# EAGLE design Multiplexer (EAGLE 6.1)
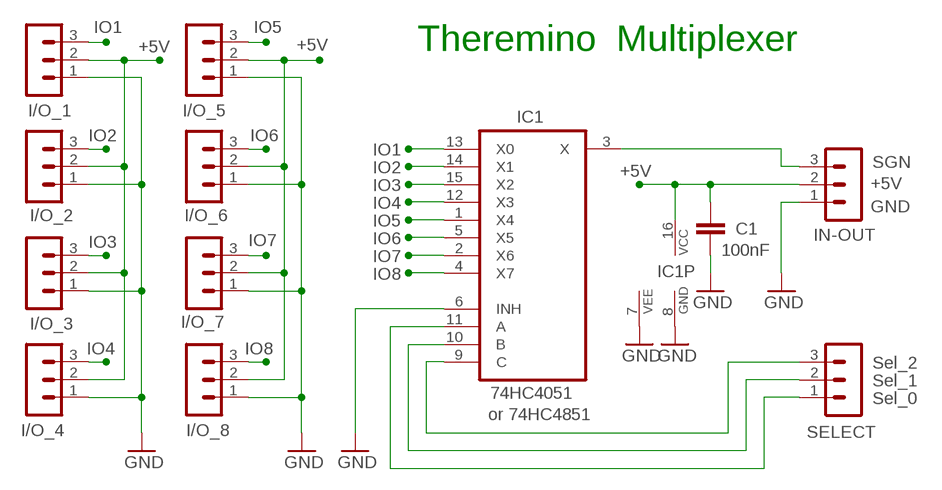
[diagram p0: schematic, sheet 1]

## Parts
C1  100nF  C-EU025-025X050  [C025-025X050]
I/O_1  MA03-1L3  [MA03-1_L3]
I/O_2  MA03-1L3  [MA03-1_L3]
I/O_3  MA03-1L3  [MA03-1_L3]
I/O_4  MA03-1L3  [MA03-1_L3]
I/O_5  MA03-1L3  [MA03-1_L3]
I/O_6  MA03-1L3  [MA03-1_L3]
I/O_7  MA03-1L3  [MA03-1_L3]
I/O_8  MA03-1L3  [MA03-1_L3]
IC1  74HC4051  4051N  [DIL16]
IN-OUT  MA03-1L3  [MA03-1_L3]
SELECT  MA03-1L3  [MA03-1_L3]

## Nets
+5V: C1.1 I/O_1.2 I/O_2.2 I/O_3.2 I/O_4.2 I/O_5.2 I/O_6.2 I/O_7.2 I/O_8.2 IC1.16(VCC) IN-OUT.2
GND: C1.2 I/O_1.1 I/O_2.1 I/O_3.1 I/O_4.1 I/O_5.1 I/O_6.1 I/O_7.1 I/O_8.1 IC1.6(INH) IC1.7(VEE) IC1.8(GND) IN-OUT.1
IO1: I/O_1.3 IC1.13(X0)
IO2: I/O_2.3 IC1.14(X1)
IO3: I/O_3.3 IC1.15(X2)
IO4: I/O_4.3 IC1.12(X3)
IO5: I/O_5.3 IC1.1(X4)
IO6: I/O_6.3 IC1.5(X5)
IO7: I/O_7.3 IC1.2(X6)
IO8: I/O_8.3 IC1.4(X7)
N$1: IC1.3(X) IN-OUT.3
N$2: IC1.11(A) SELECT.1
N$3: IC1.10(B) SELECT.2
N$4: IC1.9(C) SELECT.3

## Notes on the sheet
- Theremino | Multiplexer
- SGN
- +5V
- GND
- Sel_2
- Sel_1
- Sel_0
- or 74HC4851

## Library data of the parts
C1 = 00-LIVIO:C-EU: CAPACITOR, European symbol
I/O_1-I/O_8 IN-OUT SELECT = 03-con-lstb-M:MA03-1: PIN HEADER
IC1 = 00-LIVIO:4051: 8-channel ANALOG MULTIPLEXER

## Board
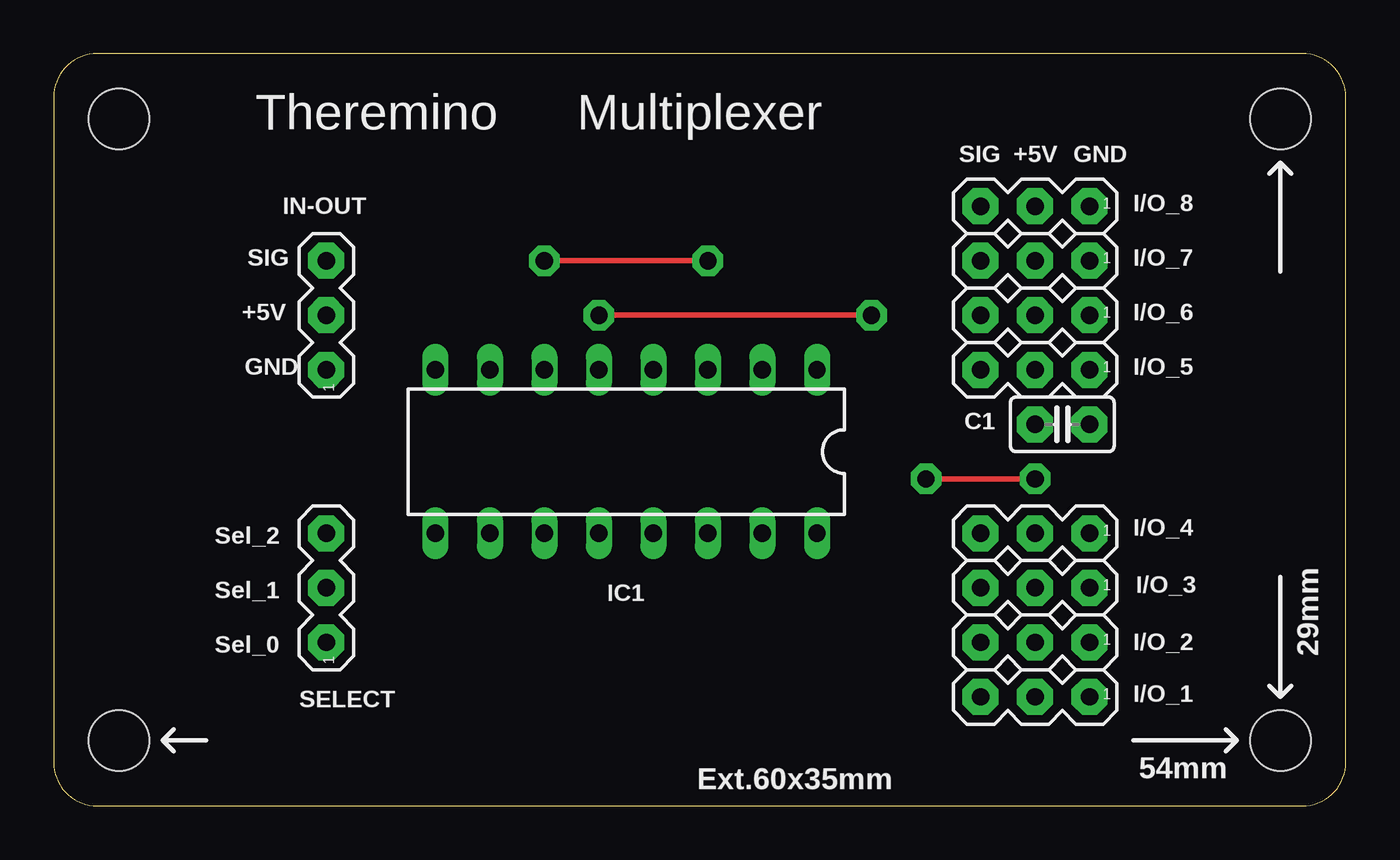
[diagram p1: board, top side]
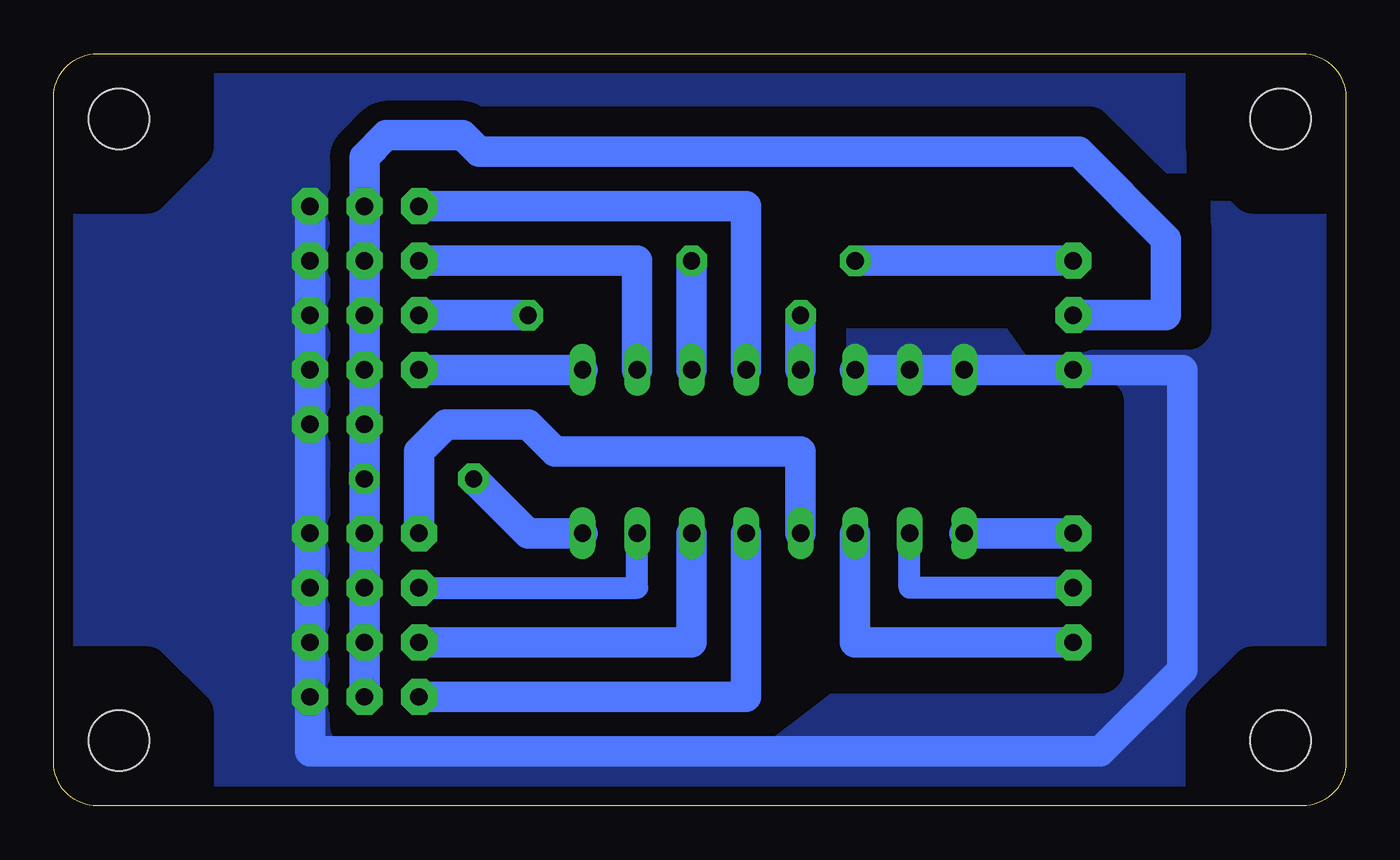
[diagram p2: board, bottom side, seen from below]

Size 60.2 x 35.05 mm. Coordinates in mm from the lower left corner, seen from the top.
Outline: 2.03,0 58.17,0 arc90 60.2,2.03 60.2,33.02 arc90 58.17,35.05 2.03,35.05 arc90 0,33.02 0,2.03 arc90 2.03,0
Copper layers (1*16): Top 0.035mm / dielectric 1.5mm / Bottom 0.035mm
Design rules: minimum track width 10mil, minimum drill 31mil, track to track 31mil, track to pad 31mil, pad to pad 31mil, via to via 31mil, smd to smd 31mil, copper to edge 31mil, drill to drill 8mil, minimum pad ring 5mil, minimum via ring 8mil, stop-mask expansion 4mil, vias tented up to drill 0mil, thermal gap 47mil
Holes 2.8 mm at 57.15,32 57.15,3.05 3.05,32 3.05,3.05
bRestrict: 23 lines

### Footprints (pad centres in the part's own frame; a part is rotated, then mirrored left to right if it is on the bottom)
C025-025X050 = drill 0.813 pad 1.676 octagon: 1 -1.27,0; 2 1.27,0
MA03-1_L3 = drill 0.813 pad 1.676 octagon: 1 -2.54,0; 2 0,0; 3 2.54,0
DIL16 = drill 0.813 long: 1 -8.89,-3.81; 2 -6.35,-3.81; 3 -3.81,-3.81; 4 -1.27,-3.81; 5 1.27,-3.81; 6 3.81,-3.81; 7 6.35,-3.81; 8 8.89,-3.81; 9 8.89,3.81; 10 6.35,3.81; 11 3.81,3.81; 12 1.27,3.81; 13 -1.27,3.81; 14 -3.81,3.81; 15 -6.35,3.81; 16 -8.89,3.81

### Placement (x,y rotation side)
C1  46.99,17.78 0 top
I/O_1  45.72,5.08 180 top
I/O_2  45.72,7.62 180 top
I/O_3  45.72,10.16 180 top
I/O_4  45.72,12.7 180 top
I/O_5  45.72,20.32 180 top
I/O_6  45.72,22.86 180 top
I/O_7  45.72,25.4 180 top
I/O_8  45.72,27.94 180 top
IC1  26.67,16.51 180 top
IN-OUT  12.7,22.86 90 top
SELECT  12.7,10.16 90 top

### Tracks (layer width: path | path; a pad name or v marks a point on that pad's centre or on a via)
+5V  (via drill 0.8 pad 1.42)
  Top 0.254: v40.64,15.24 v45.72,15.24
  Bottom 1.422: IN-OUT.2 8.38,22.86 8.38,26.42 12.45,30.48 40.39,30.48 41.15,31.24 44.7,31.24 45.72,30.23 I/O_8.2 I/O_7.2 I/O_6.2 I/O_5.2 C1.1 v45.72,15.24 I/O_4.2 I/O_3.2 I/O_2.2 I/O_1.2 | IC1.16 38.1,12.7 v40.64,15.24
GND
  Bottom 1.422: IN-OUT.1 IC1.8 IC1.7 IC1.6 IN-OUT.1 | I/O_1.1 I/O_2.1 I/O_3.1 I/O_4.1 C1.2 | I/O_8.1 I/O_7.1 I/O_6.1 I/O_5.1 C1.2 | C1.2 48.26,2.54 11.43,2.54 7.62,6.35 7.62,20.32 IN-OUT.1
  pour Bottom (isolate 0.9, no thermals): -1,-1 61.2,-1 61.2,36.05 -1,36.05
IO1
  Bottom 1.422: I/O_1.3 27.94,5.08 IC1.13
IO2
  Bottom 1.422: IC1.14 30.48,7.62 I/O_2.3
IO3
  Bottom 1.016: I/O_3.3 33.02,10.16 IC1.15
IO4
  Bottom 1.422: I/O_4.3 43.18,16.51 41.91,17.78 38.1,17.78 36.83,16.51 25.4,16.51 IC1.12
IO5
  Bottom 1.422: I/O_5.3 IC1.1
IO6  (via drill 0.8 pad 1.42)
  Top 0.254: v38.1,22.86 v25.4,22.86
  Bottom 1.422: I/O_6.3 v38.1,22.86 | v25.4,22.86 IC1.5
IO7
  Bottom 1.422: I/O_7.3 33.02,25.4 IC1.2
IO8
  Bottom 1.422: I/O_8.3 27.94,27.94 IC1.4
N$1  (via drill 0.8 pad 1.42)
  Top 0.254: v22.86,25.4 v30.48,25.4
  Bottom 1.422: IN-OUT.3 v22.86,25.4 | v30.48,25.4 IC1.3
N$2
  Bottom 1.422: IC1.11 22.86,7.62 SELECT.1
N$3
  Bottom 1.016: SELECT.2 20.32,10.16 IC1.10
N$4
  Bottom 1.422: SELECT.3 IC1.9

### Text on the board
tNames: Theremino | Multiplexer | SIG | +5V | GND | SIG | +5V | GND | Sel_2 | Sel_1 | Sel_0 | 29mm | Ext.60x35mm | 54mm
